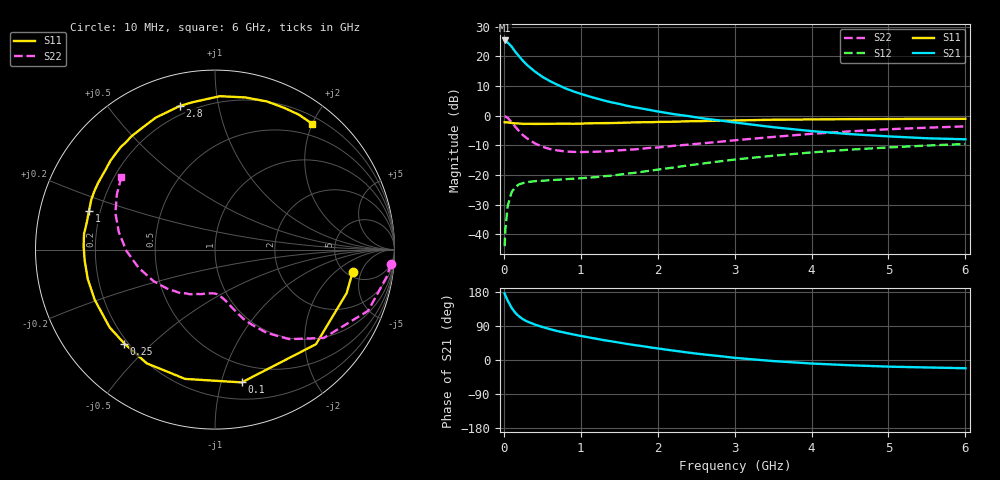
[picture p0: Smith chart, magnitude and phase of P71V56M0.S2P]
! SIEMENS Small Signal Semiconductors
! BFP196
! Si NPN RF Bipolar Junction Transistor in SOT143
! VCE = 1.5 V  IC = 6 mA
! Common Emitter S-Parameters:  May  1996
# GHz  S  MA  R  50
!  f  S11  S21  S12  S22
! GHz  MAG  ANG  MAG  ANG  MAG  ANG  MAG  ANG
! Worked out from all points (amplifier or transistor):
!   36 points, 10 MHz to 6 GHz, reference 50 ohm
!   highest |S21| = 25.4 dB at 10 MHz (marker M1)
!   |S21| within 3 dB of that: start of sweep to 126.4 MHz
!   unconditionally stable (mu >= 1): 1.033 GHz to 3.326 GHz; 5.93 GHz to end of sweep
!   at 250 MHz: K = 0.30, MSG = 20.6 dB, |S12| = -22.7 dB
!   at 1.4 GHz: K = 1.18, MAG = 9.8 dB, |S12| = -20.2 dB
!   at 6 GHz: K = 1.00, MAG = 0.5 dB, |S12| = -9.5 dB
!   S11 on the Smith chart (normalised r, x): 10 MHz: 5.61, -3.58; 100 MHz: 0.34, -1.16; 250 MHz: 0.19, -0.41; 1 GHz: 0.16, +0.15; 2.8 GHz: 0.16, +0.77; 6 GHz: 0.31, +1.99
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0.01  0.7766 -9.4  18.58 176.0  0.0063 86.9  0.9837 -4.7
0.02  0.7726 -18.2  18.06 170.1  0.0123 81.8  0.9686 -9.0
0.05  0.771 -43.1  17.14 156.8  0.0299 68.8  0.9187 -21.8
0.1  0.7547 -78.6  14.68 138.0  0.051 53.2  0.7806 -39.1
0.15  0.7394 -103.0  11.92 124.2  0.0628 42.6  0.6472 -50.4
0.2  0.7391 -121.0  9.994 114.7  0.0697 35.7  0.5469 -58.1
0.25  0.7274 -134.0  8.383 107.3  0.073 31.0  0.4681 -63.7
0.3  0.7297 -143.6  7.205 102.0  0.0755 28.6  0.416 -67.8
0.4  0.7263 -157.4  5.603 93.8  0.0786 25.0  0.3431 -73.1
0.5  0.7276 -166.9  4.538 87.2  0.0799 23.8  0.2996 -77.2
0.6  0.7288 -175.2  3.823 81.4  0.0816 23.8  0.2736 -80.9
0.7  0.7322 178.4  3.306 76.1  0.0831 23.9  0.259 -84.1
0.8  0.7349 173.1  2.894 71.8  0.0851 24.6  0.2492 -87.2
1  0.7347 162.8  2.337 63.5  0.0881 26.9  0.244 -92.6
1.1  0.7428 158.2  2.131 59.8  0.09 28.1  0.2452 -95.7
1.6  0.7647 139.6  1.468 42.4  0.1053 34.6  0.2652 -111.0
2.2  0.7909 120.5  1.066 24.9  0.1334 38.3  0.3095 -128.3
2.8  0.8239 103.7  0.833 10.4  0.1693 36.8  0.3626 -147.1
3.5  0.8552 88.2  0.64 -2.8  0.2112 31.0  0.4382 -166.8
4.5  0.8745 70.7  0.489 -13.9  0.2676 19.8  0.545 169.6
5.5  0.8854 58.0  0.416 -19.7  0.3135 7.8  0.6275 150.6
6  0.8854 52.5  0.4 -21.7  0.3337 1.3  0.6604 142.2
